FUNCTION_BLOCK FB_ProductionConfigData
VAR_INPUT
END_VAR
VAR_OUTPUT
	bError: BOOL;
	sEventClass: STRING(255);
	sEventText: STRING(255);	
	nEventID: UDINT;
END_VAR
VAR	
	nState_GetTestPara: INT;	
	nState_SetResInfo: INT;	
	nState_AddEntry: INT;
	nState_GetConfig: INT;

	
	fbPLCDBCmd: FB_PLCDBCmdEvt(sNetID:='', tTimeout:=T#5S);
	sCmd: T_MaxString;
	
	arrPara: ARRAY [0..5] OF ST_ExpParameter;
	
	_sTestNum: STRING(8);
	_stConfig: ST_Config;
	_stTest: ST_TestParameter;
	
	stTest: ST_TEST;
	
	ipResultEvt: Tc3_Eventlogger.I_TcMessage;	
END_VAR

METHOD PRIVATE _SetResultInfo : BOOL
VAR_INPUT
	nLangId: INT := 1033;
END_VAR
_SetResultInfo := FALSE;

CASE nState_SetResInfo OF
    0:
        IF ipResultEvt.RequestEventText(nLangId, sEventText, SIZEOF(sEventText)) THEN
            nState_SetResInfo := 1;
        END_IF
    1:
        IF ipResultEvt.RequestEventClassName(nLangId, sEventClass, SIZEOF(sEventClass)) THEN            
            nEventID := ipResultEvt.nEventId;

            bError := (ipResultEvt.eSeverity = TcEventSeverity.Error) OR
                     (ipResultEvt.eSeverity = TcEventSeverity.Critical);

            nState_SetResInfo:=0;
            _SetResultInfo := TRUE;         
        END_IF
END_CASE
END_METHOD

METHOD AddTestEntry : BOOL
VAR_INPUT
	sTestNum : STRING(8);
	nTypeNum : DINT;
	sTimestamp : STRING;
	sTester : STRING;
	sResult : STRING; 
END_VAR
AddTestEntry := FALSE;

arrPara[0].sParaName := 'TestNum';
arrPara[0].eParaType := Tc3_Database.E_ExpParameterType.STRING_;
arrPara[0].nParaSize := 8;

arrPara[1].sParaName := 'TypeNum';
arrPara[1].eParaType := Tc3_Database.E_ExpParameterType.Int32;
arrPara[1].nParaSize := 4;

arrPara[2].sParaName := 'Timestamp';
arrPara[2].eParaType := Tc3_Database.E_ExpParameterType.STRING_;
arrPara[2].nParaSize := 81;

arrPara[3].sParaName := 'Tester';
arrPara[3].eParaType := Tc3_Database.E_ExpParameterType.STRING_;
arrPara[3].nParaSize := 81;

arrPara[4].sParaName := 'Result';
arrPara[4].eParaType := Tc3_Database.E_ExpParameterType.STRING_;
arrPara[4].nParaSize := 81;

arrPara[5].sParaName := 'Test';
arrPara[5].eParaType := Tc3_Database.E_ExpParameterType.XMLTAGName;
arrPara[5].nParaSize := 0;

sCmd := 'XPATH_ADD<ATTR>#ProductionConfig/Tests';

stTest.sTestNum := sTestNum;
stTest.nTypeNum := nTypeNum;
stTest.sTimestamp := sTimestamp;
stTest.sTester := sTester;
stTest.sResult := sResult;

CASE nState_AddEntry OF
	0:
		IF fbPLCDBCmd.Execute(
			hDBID:= 2, 
			pExpression:= ADR(sCmd), 
			cbExpression:= SIZEOF(sCmd), 
			pData:= ADR(stTest), 
			cbData:= SIZEOF(stTest), 
			pParameter:= ADR(arrPara), 
			cbParameter:= SIZEOF(arrPara)) THEN	
			
			ipResultEvt := fbPLCDBCmd.ipTcResult;
			nState_AddEntry:= 100;
		END_IF
	100:
		IF _SetResultInfo(1033) THEN
			nState_AddEntry:= 0;
			AddTestEntry := TRUE;			
		END_IF	
END_CASE
END_METHOD

METHOD GetConfig : BOOL
VAR_INPUT
	nTypeNum : DINT;
END_VAR
VAR_OUTPUT
	stConfig : ST_Config;
END_VAR
GetConfig := FALSE;

arrPara[0].sParaName := 'rLength';
arrPara[0].eParaType := Tc3_Database.E_ExpParameterType.Float32;
arrPara[0].nParaSize := 4;

arrPara[1].sParaName := 'rWidth';
arrPara[1].eParaType := Tc3_Database.E_ExpParameterType.Float32;
arrPara[1].nParaSize := 4;

arrPara[2].sParaName := 'rHeight';
arrPara[2].eParaType := Tc3_Database.E_ExpParameterType.Float32;
arrPara[2].nParaSize := 4;

arrPara[3].sParaName := 'iQuantity';
arrPara[3].eParaType := Tc3_Database.E_ExpParameterType.Int32;
arrPara[3].nParaSize := 4;

arrPara[4].sParaName := 'iCounter';
arrPara[4].eParaType := Tc3_Database.E_ExpParameterType.Int32;
arrPara[4].nParaSize := 4;

sCmd := CONCAT(CONCAT('XPATH_SEL<SUBTAG>#ProductionConfig/Config[@TypeNum = ', DINT_TO_STRING(nTypeNum)), ']');

CASE nState_GetConfig OF
	0:
		IF fbPLCDBCmd.ExecuteDataReturn(
			hDBID:= 1, 
			pExpression:= ADR(sCmd), 
			cbExpression:= SIZEOF(sCmd), 
			pData:= 0, 
			cbData:= 0, 
			pParameter:= ADR(arrPara), 
			cbParameter:= SIZEOF(arrPara[0])*5, 
			nStartIndex:= 0, 
			nRecordCount:= 1, 
			pReturnData:= ADR(_stConfig), 
			cbReturnData:= SIZEOF(_stConfig), 
			pRecords:= 0) THEN	
						
			ipResultEvt := fbPLCDBCmd.ipTcResult;
			nState_GetConfig := 100;	
		END_IF
	100:
		IF _SetResultInfo(1033) THEN
			GetConfig := TRUE;
			
			stConfig := _stConfig;
			
			nState_GetConfig := 0;	
		END_IF
END_CASE
END_METHOD

METHOD GetTestParameter : BOOL
VAR_INPUT
	nTypeNum : DINT;
END_VAR
VAR_OUTPUT	
	sTestNum : STRING(8);
	stTestPara: ST_TestParameter;	
END_VAR
GetTestParameter := FALSE;

CASE nState_GetTestPara OF
	0:
		arrPara[0].sParaName := 'Test';
		arrPara[0].eParaType := Tc3_Database.E_ExpParameterType.STRING_;
		arrPara[0].nParaSize := 8;

		sCmd := CONCAT(CONCAT('XPATH_SEL<ATTR>#ProductionConfig/Config[@TypeNum = ', DINT_TO_STRING(nTypeNum)), ']');
		
		IF fbPLCDBCmd.ExecuteDataReturn(
			hDBID:= 1, 
			pExpression:= ADR(sCmd), 
			cbExpression:= SIZEOF(sCmd), 
			pData:= 0, 
			cbData:= 0, 
			pParameter:= ADR(arrPara), 
			cbParameter:= SIZEOF(arrPara[0]), 
			nStartIndex:= 0, 
			nRecordCount:= 1, 
			pReturnData:= ADR(_sTestNum), 
			cbReturnData:= SIZEOF(_sTestNum), 
			pRecords:= 0) THEN	
			
			IF fbPLCDBCmd.bError THEN
				ipResultEvt := fbPLCDBCmd.ipTcResult;
				nState_GetTestPara := 100;
			ELSE
				nState_GetTestPara := 1;
			END_IF
		END_IF		
	1:
		arrPara[0].sParaName := 'MaxTemp';
		arrPara[0].eParaType := Tc3_Database.E_ExpParameterType.Float32;
		arrPara[0].nParaSize := 4;
		
		arrPara[1].sParaName := 'MinTemp';
		arrPara[1].eParaType := Tc3_Database.E_ExpParameterType.Float32;
		arrPara[1].nParaSize := 4;
		
		arrPara[2].sParaName := 'MaxPSI';
		arrPara[2].eParaType := Tc3_Database.E_ExpParameterType.Int32;
		arrPara[2].nParaSize := 4;
		
		sCmd := CONCAT(CONCAT('XPATH_SEL<SUBTAG>#ProductionConfig/TestParameter/Test[@Num = $'', _sTestNum), '$']');
		
		IF fbPLCDBCmd.ExecuteDataReturn(
			hDBID:= 2, 
			pExpression:= ADR(sCmd), 
			cbExpression:= SIZEOF(sCmd), 
			pData:= 0, 
			cbData:= 0, 
			pParameter:= ADR(arrPara), 
			cbParameter:= SIZEOF(arrPara[0])*3, 
			nStartIndex:= 0, 
			nRecordCount:= 1, 
			pReturnData:= ADR(_stTest), 
			cbReturnData:= SIZEOF(_stTest), 
			pRecords:= 0) THEN	
						
			ipResultEvt := fbPLCDBCmd.ipTcResult;
			
			nState_GetTestPara := 100;	
		END_IF
	100:
		IF _SetResultInfo(1033) THEN
			nState_GetTestPara := 0;
			
			stTestPara := _stTest;			
			sTestNum := _sTestNum;
			
			GetTestParameter := TRUE;
		END_IF
END_CASE
END_METHOD

END_FUNCTION_BLOCK
